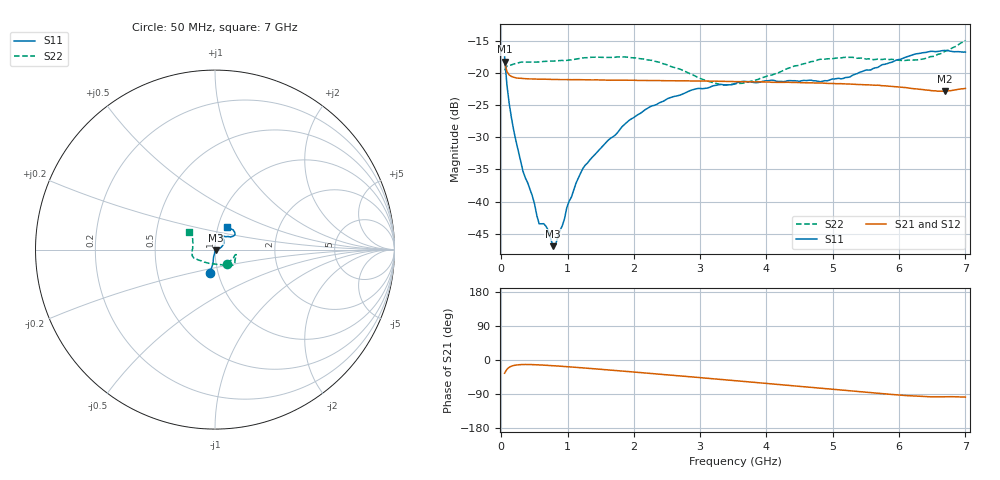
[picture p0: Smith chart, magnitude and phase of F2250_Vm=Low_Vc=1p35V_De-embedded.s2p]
! Integrated Device Technology
! Corporate Headquarters
! 6024 Silver Creek Valley Road
! San Jose, CA 95138  USA
! Phone:  1-408-284-8200
! Toll Free:  1-800-223-1366
! Webpage:  http://www.idt.com/
! Timing and RF Division
! 515 Groton Road, Suite 102
! Westford, MA 01886-6024
! Device:  F2250
! Description: Voltage Variable RF Attenuator
! Frequency:  50.0 -  6000.00 MHz
! Package:  3x3 mm Thin QFN Plastic Package: 16 pin
! Ports:  2 RF, 3 DC
!  Pin  1  = GND
!  Pin  2  = NC
!  Pin  3  = RF1  = Port 1
!  Pin  4  = NC
!  Pin  5  = GND
!  Pin  6  = GND
!  Pin  7  = GND
!  Pin  8  = GND
!  Pin  9  = NC
!  Pin 10  = RF2  = Port 2
!  Pin 11  = NC
!  Pin 12  = GND
!  Pin 13  = GND
!  Pin 14  = VCNTRL
!  Pin 15  = VDD
!  Pin 16  = VMODE
! Vcntrl:  1.350 Volts
! Vmode:  +0.000 Volts
! Vdd:  +3.30  Volts
! Current:  1.192 mA
! Data:  The device was measured on a the F2250 evaluation board which has
!  individual transmission lines to the RF pins.  Data was collected
!  using a calibrated network analyzer.  The evaluation board was
!  de-embedded using a TRL calibration technique.
!  The reference plane is the edge of the package pin.
! Misc:  SN 10
!  Action Tracker AT0258
! Date Measured:  2014-11-26
! Date:  2015-10-15  MJV
! Note:
!  Integrated Device Technology supplies this data as a sample of measured
!  data at the package pin for this product.  Your particular data for this
!  product may vary.
!  Data was taken at 25 degrees C.
!  Integrated Device Technology reserves the right to change this data at anytime.
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# GHz S dB R 50
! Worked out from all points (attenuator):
!   201 points, 50 MHz to 7 GHz, reference 50 ohm
!   highest |S21| = -18.31 dB at 50 MHz (marker M1); lowest = -22.9 dB at 6.687 GHz (marker M2)
!   lowest |S11| = -46.9 dB at 779.8 MHz (marker M3), VSWR 1.01, Z = 50.3 - j0.295 ohm
!   |S11| at or under -10 dB: start of sweep to end of sweep
!   |S22| runs from -21.9 to -15.0 dB; largest |S21 - S12| = 0.00037
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0.05  -17.55 -102.6  -18.31 -34.8  -18.30 -34.8  -19.64 -48.7
0.08475  -21.87 -98.2  -19.84 -24.5  -19.84 -24.5  -18.97 -24.9
0.15425  -27.07 -100.8  -20.58 -16.2  -20.57 -16.2  -18.78 -15.1
0.328  -35.32 -96.5  -20.89 -11.9  -20.89 -11.9  -18.34 -13.2
0.467  -39.09 -96.4  -20.96 -12.1  -20.96 -12.1  -18.36 -14.7
0.57125  -43.47 -81.1  -20.99 -12.9  -20.99 -12.9  -18.33 -17.2
0.6755  -43.86 -66.1  -21.01 -13.9  -21.00 -13.9  -18.22 -19.5
0.77975  -46.94 -40.7  -21.05 -15.1  -21.04 -15.1  -18.20 -22.1
0.8145  -46.80 -31.6  -21.04 -15.5  -21.03 -15.5  -18.17 -23.1
0.9535  -42.68 -24.7  -21.06 -17.1  -21.04 -17.1  -18.16 -26.4
0.98825  -40.94 -18.6  -21.05 -17.6  -21.06 -17.6  -18.08 -26.9
1.2315  -34.85 2.9  -21.10 -20.8  -21.09 -20.8  -17.70 -31.6
1.9265  -27.41 24.6  -21.16 -30.7  -21.15 -30.7  -17.62 -41.1
2.37825  -24.70 34.8  -21.20 -37.3  -21.22 -37.3  -18.35 -48.0
3.14275  -22.27 56.1  -21.30 -48.7  -21.29 -48.7  -21.39 -77.1
3.525  -21.68 66.5  -21.39 -54.5  -21.38 -54.5  -21.73 -104.0
4.7065  -21.24 69.4  -21.57 -72.7  -21.58 -72.7  -18.24 -156.4
5.22775  -20.72 52.7  -21.75 -80.9  -21.74 -80.9  -17.60 -165.3
5.85325  -18.46 37.3  -22.10 -90.3  -22.11 -90.4  -17.96 -177.5
6.305  -17.00 38.4  -22.57 -96.0  -22.57 -96.0  -17.96 166.3
6.68725  -16.53 47.2  -22.88 -97.0  -22.86 -97.0  -16.70 149.7
7  -16.79 62.7  -22.43 -97.8  -22.41 -98.0  -14.99 145.7
